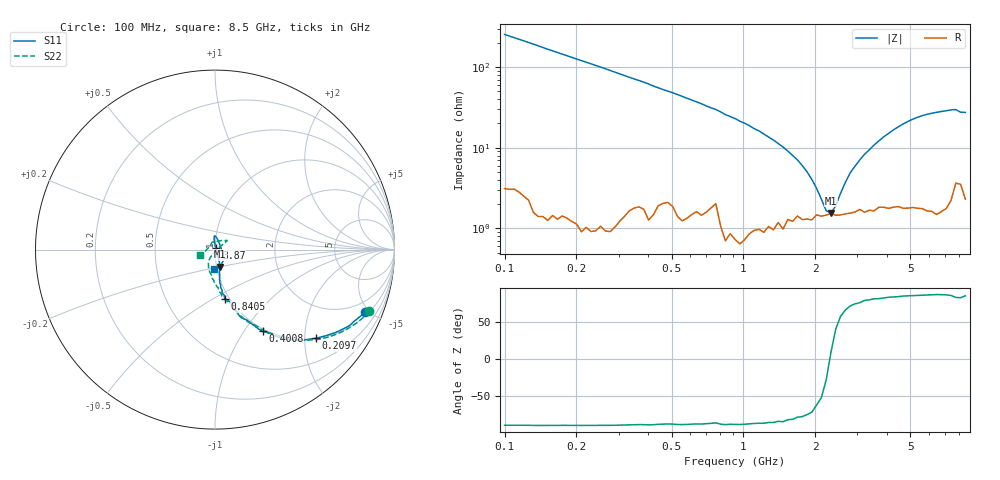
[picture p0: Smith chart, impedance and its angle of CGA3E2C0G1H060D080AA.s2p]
! S-parameter Generated by TDK Corporation
! Copyright(C) 2015 TDK Corporation.
! All Rights Reserved.
! TDK P/N: CGA3E2C0G1H060D080AA (Multilayer Ceramic Chip Capacitors)
! Property: C=6pF
! Size(LxWxT): 1.6x0.8x0.8mm, 0.063x0.031x0.031inches
! Model Type: s2p (Touchstone File Format Version 1.0)
! Frequency: DC=Yes Start=100MHz Stop=8500MHz 98points Log-sweep
! Note:
! Model Generated on Jun. 23, 2015
! Hash(MD5):
! Port Assignments:
!  1 ---| |--- 2
! Applicable Conditions:
!  Temperature = 25 degC
!  DC Bias Voltage = 0 V
!  Small Signal Operation
! Terms and conditions regarding TDK Simulation Models
! (1)This simulation model is being provided solely for informational purposes. Please refer to the specifications of the products in terms of detailed characteristics of such products.
! (2)In no event shall TDK Corporation of any of its subsidiaries be liable for any loss or damage arising, directly or indirectly,
!  From any information contained in this simulation model, including, but not limited to loss or damages arising from any inaccuracies, omissions or errors in connection with such information.
! (3)Any and all copyrights on this simulation model are owned by TDK Corporation.
!  Duplication or redistribution of this simulation model without prior written permission from TDK Corporation is prohibited.
! (4)This simulation model is subject to any modification or change without any prior notice.
! (5)Neither TDK Corporation nor any of its subsidiaries shall make any warranty, express or implied,
!  Including but not limited to the correctness, implied warranties of merchantability and fitness for a particular purpose with respect to this simulation models.
! (6)The use of this simulation model shall be deemed to have consented to the terms and conditions hereof.
# MHz S MA R 50
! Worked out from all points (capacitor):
!   97 points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, 100 MHz to 8.5 GHz, reference 50 ohm
!   read as one part in series: C = 6.24 pF near 100 MHz
!   lowest |Z| = 1.55 ohm at 2.326 GHz (marker M1)
!   series resonance near 2.301 GHz, so ESL is about 770 pH
!   S11 on the Smith chart (normalised r, x): 100 MHz: 1.21, -4.74; 209.7 MHz: 1.01, -2.26; 400.8 MHz: 0.97, -1.22; 840.5 MHz: 0.96, -0.57; 3.87 GHz: 1.02, +0.02; 8.5 GHz: 0.97, -0.21
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100  0.9069 -22.5  0.3595 67.3  0.3592 67.3  0.9257 -21.8
209.6862  0.7476 -41.3  0.6224 49.2  0.6228 49.1  0.7686 -40.4
400.8145  0.5282 -59.6  0.8297 30.1  0.831 30.1  0.5307 -58.9
554.1537  0.4065 -68.9  0.8877 21.5  0.8889 21.5  0.4125 -67.6
840.4526  0.2798 -78.3  0.9441 12.0  0.9441 11.9  0.2845 -78.1
1533.871  0.1599 -80.6  0.9652 1.0  0.9659 1.0  0.1552 -95.3
2326.332  0.09807 -74.1  0.9702 -5.8  0.9696 -5.8  0.09929 -111.1
2931.989  0.06079 -70.0  0.9702 -9.8  0.971 -9.9  0.06283 -120.1
3368.656  0.03142 -62.6  0.9718 -12.5  0.9717 -12.5  0.03556 -116.0
3528.213  0.01585 -54.9  0.9708 -13.4  0.9704 -13.4  0.02347 -112.5
3695.327  0.01022 -39.2  0.9703 -14.4  0.9691 -14.4  0.01185 -85.1
3870.357  0.01331 54.6  0.9693 -15.4  0.9696 -15.3  0.008901 -29.0
4053.677  0.01926 88.1  0.9697 -16.5  0.9684 -16.4  0.01964 20.1
4245.68  0.0337 89.8  0.9683 -17.5  0.9673 -17.5  0.03189 31.1
4446.777  0.04387 94.4  0.9666 -18.7  0.9665 -18.6  0.0463 32.1
5109.044  0.07202 93.2  0.9648 -22.3  0.9632 -22.3  0.0786 36.2
5869.945  0.07266 87.0  0.9623 -26.4  0.9616 -26.3  0.07856 39.9
7063.606  0.0354 10.6  0.9596 -32.8  0.9565 -32.7  0.04506 91.1
7398.175  0.04894 -25.7  0.9537 -34.7  0.9546 -34.8  0.04364 112.8
7748.59  0.07638 -50.4  0.9355 -36.7  0.9368 -36.5  0.03444 141.3
8115.603  0.1025 -76.9  0.9355 -37.2  0.9371 -37.1  0.06046 -167.0
8500  0.1095 -92.2  0.9478 -39.2  0.9488 -38.9  0.09149 -159.2
